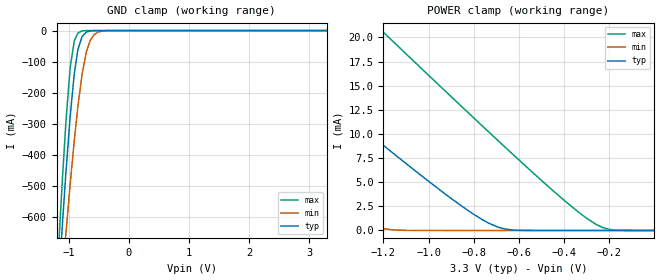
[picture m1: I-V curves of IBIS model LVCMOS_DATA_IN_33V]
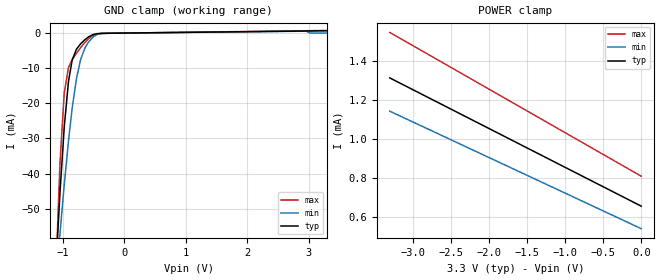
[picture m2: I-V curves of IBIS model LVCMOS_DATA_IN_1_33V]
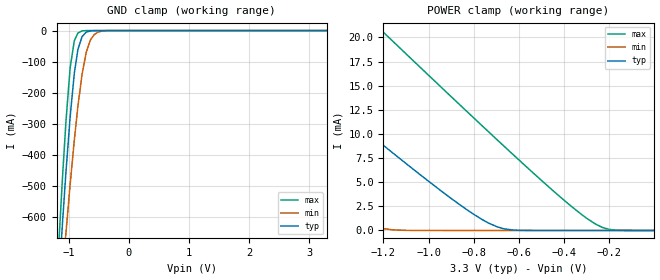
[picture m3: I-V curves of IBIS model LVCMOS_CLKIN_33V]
|   National Semiconductor
|   DS90UH925AQ-Q1
[IBIS Ver]   4.2
[File name]   ds90uh925aq_q1.ibs
[File Rev]   1.1
[Date]   05/04/2010 Rev. 1.1
|   02/03/2011 Rev. 1.0
[Source]   SPICE to IBIS Translation
[Notes]
CML Outputs are NOT SUPPORTED in this version of the IBIS model
The following IBIS parser notes and warnings have been reviewed and are
considered very minor ans should not cause any modeling issues:
WARNING (line 4219) - GND Clamp Minimum data is non-monotonic
WARNING -
   Model LVCMOS_DATA_IN_33V: POWER Clamp : Maximum value never becomes zero
WARNING (line 4437) - GND Clamp Minimum data is non-monotonic
WARNING -
   Model LVCMOS_DATA_IN_1_33V: POWER Clamp : Typical value never becomes zero
WARNING -
   Model LVCMOS_DATA_IN_1_33V: POWER Clamp : Minimum value never becomes zero
WARNING -
   Model LVCMOS_DATA_IN_1_33V: POWER Clamp : Maximum value never becomes zero
WARNING (line 4654) - GND Clamp Minimum data is non-monotonic
WARNING -
   Model LVCMOS_CLKIN_33V: POWER Clamp : Maximum value never becomes zero
WARNING (line 4872) - GND Clamp Minimum data is non-monotonic
WARNING (line 5090) - GND Clamp Minimum data is non-monotonic
WARNING -
   Model LVCMOS_PWDN_3325V_33V: POWER Clamp : Typical value never becomes zero
WARNING -
   Model LVCMOS_PWDN_3325V_33V: POWER Clamp : Minimum value never becomes zero
WARNING -
   Model LVCMOS_PWDN_3325V_33V: POWER Clamp : Maximum value never becomes zero
WARNING (line 5308) - GND Clamp Minimum data is non-monotonic
WARNING (line 5525) - GND Clamp Minimum data is non-monotonic
WARNING (line 5743) - GND Clamp Minimum data is non-monotonic
WARNING -
   Model LVCMOS_DATA_IN_1_18V: POWER Clamp : Typical value never becomes zero
WARNING -
   Model LVCMOS_DATA_IN_1_18V: POWER Clamp : Minimum value never becomes zero
WARNING -
   Model LVCMOS_DATA_IN_1_18V: POWER Clamp : Maximum value never becomes zero
WARNING (line 5959) - GND Clamp Minimum data is non-monotonic
WARNING (line 6177) - GND Clamp Minimum data is non-monotonic
WARNING -
   Model LVCMOS_PWDN_3325V_18V: POWER Clamp : Typical value never becomes zero
WARNING -
   Model LVCMOS_PWDN_3325V_18V: POWER Clamp : Maximum value never becomes zero
WARNING (line 6395) - GND Clamp Minimum data is non-monotonic
WARNING (line 6613) - GND Clamp Minimum data is non-monotonic
Errors  : 0
Warnings: 25
File Passed
[Disclaimer]
(C) Copyright National Semiconductor Corporation 2011
   All rights reserved
National Semiconductor Corporation hereby grants the
user of this IBIS model a non-exclusive, nontransferable
license to use this IBIS model under the following terms.
Before using this IBIS model, the user should read this
license.  If the user does not accept these terms,  the
IBIS model should be returned to National within 30 days.
The user is granted this license only to use the
IBIS model and is not granted rights to sell, load, rent,
lease or license the IBIS model in whole or in part, or in
modified form to anyone other than user. User may modify
the IBIS model to suit its specific applications but rights
to derivative works and such modifications shall belong to
National.
This IBIS model is provided on an "AS IS" basis and
National makes absolutely no warranty with respect to the
information contained herein.NATIONAL DISCLAIMS AND CUSTOMER
WAIVES ALL WARRANTIES, EXPRESS OR IMPLIED, INCLUDING
WARRANTIES OF MERCHANTABILITY OR FITNESS FOR A PARTICULAR
PURPOSE. The entire risk as to quality and performance is
with the Customer. ACCORDINGLY, IN NO EVENT SHALL THE
COMPANY BE LIABLE FOR ANY DAMAGES, WHETHER IN CONTRACT OR
TORT,INCLUDING ANY LOST PROFITS OR OTHER INCIDENTAL,
CONSEQUENTIAL, EXEMPLARY, OR PUNITIVE DAMAGES ARISING OUT
OF THE USE OR APPLICATION OF THE IBIS model provided in
this package.Further, National reserves the right to make
changes without notice to any product herein to improve
reliability, function, or design. National does not convey
any license under patent rights or any other intellectual
property rights, including those of third parties.
National is not obligated to provide maintenance or support
for the licensed IBIS model.
[Copyright]   Copyright 2011, National Semiconductor, All Rights Reserved
[Component]   DS90UH925AQ-Q1
Si_location   Pin
Timing_location   Pin
[Manufacturer]   National Semiconductor
[Package]
R_pkg   0m   0m   0m
L_pkg   0n   0n   0n
C_pkg   0p   0p   0p
[PIN]   signal_name   model_name   R_pin   L_pin   C_pin
1   B6   LVCMOS_DATA_IN
2   B7   LVCMOS_DATA_IN
3   HS   LVCMOS_DATA_IN_1
4   VS   LVCMOS_DATA_IN_1
5   DE   LVCMOS_DATA_IN
6   IDx   NC
7   CAPL12   NC
8   SCL   NC
9   SDA   NC
10   PCLK   LVCMOS_CLKIN
11   I2S_DA   LVCMOS_IO_IN
12   I2S_WC   LVCMOS_IO_IN
13   GPO_REG8   LVCMOS_IO_IN
14   CAPP12   NC
15   RES0   NC
16   REM_INTB   LVCMOS_IO_IN
17   CAPHS12   NC
18   RES1   NC
19   DOUTm   NC
20   DOUTp   NC
21   PDB   LVCMOS_PWDN_3325V
22   VDD33   POWER
23   CMF   NC
24   MODE_SEL   NC
25   R0   LVCMOS_IO_IN_1
26   R1   LVCMOS_IO_IN_1
27   R2   LVCMOS_DATA_IN
28   R3   LVCMOS_DATA_IN
29   R4   LVCMOS_DATA_IN
30   VDDIO   POWER
31   INTB   NC
32   R5   LVCMOS_DATA_IN
33   R6   LVCMOS_DATA_IN
34   R7   LVCMOS_DATA_IN
35   GO   LVCMOS_IO_IN
36   G1   LVCMOS_IO_IN
37   G2   LVCMOS_DATA_IN
38   G3   LVCMOS_DATA_IN
39   G4   LVCMOS_DATA_IN
40   G5   LVCMOS_DATA_IN
41   G6   LVCMOS_DATA_IN
42   G7   LVCMOS_DATA_IN
43   B0   LVCMOS_IO_IN
44   B1   LVCMOS_IO_IN
45   B2   LVCMOS_DATA_IN
46   B3   LVCMOS_DATA_IN
47   B4   LVCMOS_DATA_IN
48   B5   LVCMOS_DATA_IN
DAP   GND   GND
|   Model Selectors
[Model Selector]  LVCMOS_DATA_IN
LVCMOS_DATA_IN_33V   3.3V input
LVCMOS_DATA_IN_18V   1.8V input
[Model Selector]  LVCMOS_DATA_IN_1
LVCMOS_DATA_IN_1_33V   3.3V input
LVCMOS_DATA_IN_1_18V   1.8V input
[Model Selector]  LVCMOS_CLKIN
LVCMOS_CLKIN_33V   3.3V input
LVCMOS_CLKIN_18V   1.8V input
[Model Selector]  LVCMOS_IO_IN
LVCMOS_IO_IN_33V   3.3V input
LVCMOS_IO_IN_18V   1.8V input
[Model Selector]  LVCMOS_PWDN_3325V
LVCMOS_PWDN_3325V_33V   3.3V input
LVCMOS_PWDN_3325V_18V   1.8V input
[Model Selector]  LVCMOS_IO_IN_1
LVCMOS_IO_IN_1_33V   3.3V input
LVCMOS_IO_IN_1_18V   1.8V input
[Define Package Model] llp48_v2_ds90uh925
[Manufacturer]  Unknown
[OEM]  Unknown
[Description]  Ansoft Q3D Extractor Pkg model - buildsheet DS90UB925QSQ
[Number Of Pins]  48
[Pin Numbers]
49   | 49 = DAP
1   | 1 = L1
2   | 2 = L2
3   | 3 = L3
4   | 4 = L4
5   | 5 = L5
6   | 6 = L6
7   | 7 = L7
8   | 8 = L8
9   | 9 = L9
10   | 10 = L10
11   | 11 = L11
12   | 12 = L12
13   | 13 = L13
14   | 14 = L14
15   | 15 = L15
17   | 17 = L17
18   | 18 = L18
19   | 19 = L19
20   | 20 = L20
21   | 21 = L21
22   | 22 = L22
23   | 23 = L23
24   | 24 = L24
25   | 25 = L25
26   | 26 = L26
27   | 27 = L27
28   | 28 = L28
29   | 29 = L29
30   | 30 = L30
31   | 31 = L31
32   | 32 = L32
33   | 33 = L33
34   | 34 = L34
35   | 35 = L35
36   | 36 = L36
37   | 37 = L37
38   | 38 = L38
39   | 39 = L39
40   | 40 = L40
41   | 41 = L41
42   | 42 = L42
43   | 43 = L43
44   | 44 = L44
45   | 45 = L45
46   | 46 = L46
47   | 47 = L47
48   | 48 = L48
[Model Data]
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[End Model Data]
[End Package Model]
| Models and submodels in the file (12): LVCMOS_DATA_IN_33V (Input), LVCMOS_DATA_IN_1_33V (Input), LVCMOS_CLKIN_33V (Input), LVCMOS_IO_IN_33V (Input), LVCMOS_PWDN_3325V_33V (Input), LVCMOS_IO_IN_1_33V (Input), LVCMOS_DATA_IN_18V (Input), LVCMOS_DATA_IN_1_18V (Input), LVCMOS_CLKIN_18V (Input), LVCMOS_PWDN_3325V_18V (Input), LVCMOS_IO_IN_1_18V (Input), LVCMOS_IO_IN_18V (Input)
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[Model] LVCMOS_DATA_IN_33V
Model_type Input
Vinh = 2.0V
Vinl = 0.8V
C_comp   6.98pF   6.05pF   8.06pF
[Voltage Range]   3.3V   2.97V   3.63V
[Temperature Range]   25.0   130.0   -40.0
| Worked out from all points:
|   GND clamp passes 1 mA (typ) near -0.64 V on its own axis
|   POWER clamp passes 1 mA (typ) near -0.75 V on its own axis
[GND Clamp]
-3.3V     -7.729A    -6.4A      -8.836A
-1.171V   -833.9mA   -960.9mA   -719.2mA
-1.102V   -623.3mA   -790.6mA   -477.4mA
-1.043V   -454.3mA   -650.1mA   -290.9mA
-973.5mV  -277.4mA   -494.8mA   -119.9mA
-904.2mV  -136.9mA   -352.1mA   -32.52mA
-844.8mV  -61.18mA   -243.7mA   -7.904mA
-775.5mV  -19.33mA   -140.4mA   -1.013mA
-706.2mV  -4.959mA   -70.01mA   -78.98uA
-636.9mV  -979uA     -30.5mA    -10.61uA
-438.9mV  -5.524uA   -1.421mA   -493.3nA
3.293V    492.2nA    0A         630.2nA
[POWER Clamp]
-3.3V     49.92mA    32.15mA    67.97mA
-2.597V   36.03mA    20.71mA    52.03mA
-1.835V   21.06mA    8.532mA    34.8mA
-1.795V   20.29mA    7.916mA    33.91mA
-1.399V   12.62mA    2.095mA    25mA
-1.201V   8.841mA    190.7uA    20.57mA
-864.6mV  2.717mA    1.43uA     13.09mA
-696.3mV  373.5uA    1.191uA    9.393mA
-399.3mV  1.092uA    858nA      3.115mA
-260.7mV  851.6nA    730.9nA    661uA
-201.3mV  761.3nA    681.9nA    114.6uA
-3.3mV    503.4nA    542nA      1.401uA
[Model] LVCMOS_DATA_IN_1_33V
Model_type Input
Vinh = 2.0V
Vinl = 0.8V
C_comp   3.35pF   3.347pF   3.362pF
[Voltage Range]   3.3V   2.97V   3.63V
[Temperature Range]   25.0   130.0   -40.0
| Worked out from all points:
|   GND clamp passes 1 mA (typ) near -0.57 V on its own axis
|   POWER clamp passes 1 mA (typ) near -1.73 V on its own axis
[GND Clamp]
-3.3V     -1.028A    -640.2mA   -1.808A
-1.102V   -64.66mA   -69.85mA   -64.75mA
-1.043V   -45.56mA   -57.14mA   -37.08mA
-973.5mV  -26.84mA   -43.23mA   -17.1mA
-904.2mV  -13.75mA   -30.69mA   -9.794mA
-844.8mV  -7.703mA   -21.46mA   -7.561mA
-775.5mV  -4.629mA   -13.03mA   -5.756mA
-706.2mV  -3.04mA    -7.476mA   -4.121mA
-636.9mV  -1.873mA   -4.26mA    -2.642mA
-508.2mV  -451.6uA   -1.142mA   -662.5uA
-240.9mV  -48.27uA   -48.43uA   -54.28uA
3.293V    654.7uA    0A         733.9uA
[POWER Clamp]
-3.3V     1.312mA    1.142mA    1.544mA
-3.231V   1.298mA    1.129mA    1.529mA
-3.191V   1.29mA     1.122mA    1.52mA
-3.3mV    656.6uA    541.5uA    809.7uA
[Model] LVCMOS_CLKIN_33V
Model_type Input
Vinh = 2.0V
Vinl = 0.8V
C_comp   6.98pF   6.05pF   8.06pF
[Voltage Range]   3.3V   2.97V   3.63V
[Temperature Range]   25.0   130.0   -40.0
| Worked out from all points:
|   GND clamp passes 1 mA (typ) near -0.64 V on its own axis
|   POWER clamp passes 1 mA (typ) near -0.75 V on its own axis
[GND Clamp]
-3.3V     -7.729A    -6.4A      -8.836A
-1.171V   -833.8mA   -960.9mA   -719.2mA
-1.102V   -623.2mA   -790.6mA   -477.4mA
-1.043V   -454.2mA   -650.1mA   -290.9mA
-973.5mV  -277.4mA   -494.8mA   -119.9mA
-904.2mV  -136.9mA   -352.1mA   -32.52mA
-844.8mV  -61.17mA   -243.7mA   -7.904mA
-775.5mV  -19.32mA   -140.4mA   -1.013mA
-706.2mV  -4.959mA   -70.01mA   -78.98uA
-636.9mV  -979uA     -30.5mA    -10.61uA
-438.9mV  -5.517uA   -1.421mA   -493.3nA
3.293V    492.2nA    0A         630.2nA
[POWER Clamp]
-3.3V     49.92mA    32.15mA    67.97mA
-2.597V   36.03mA    20.71mA    52.03mA
-1.835V   21.06mA    8.532mA    34.8mA
-1.795V   20.29mA    7.916mA    33.91mA
-1.399V   12.62mA    2.095mA    25mA
-1.201V   8.841mA    190.7uA    20.57mA
-864.6mV  2.717mA    1.43uA     13.09mA
-696.3mV  373.5uA    1.191uA    9.393mA
-399.3mV  1.092uA    858.1nA    3.115mA
-260.7mV  851.6nA    730.9nA    661uA
-201.3mV  761.3nA    681.9nA    114.6uA
-3.3mV    503.4nA    542nA      1.401uA
